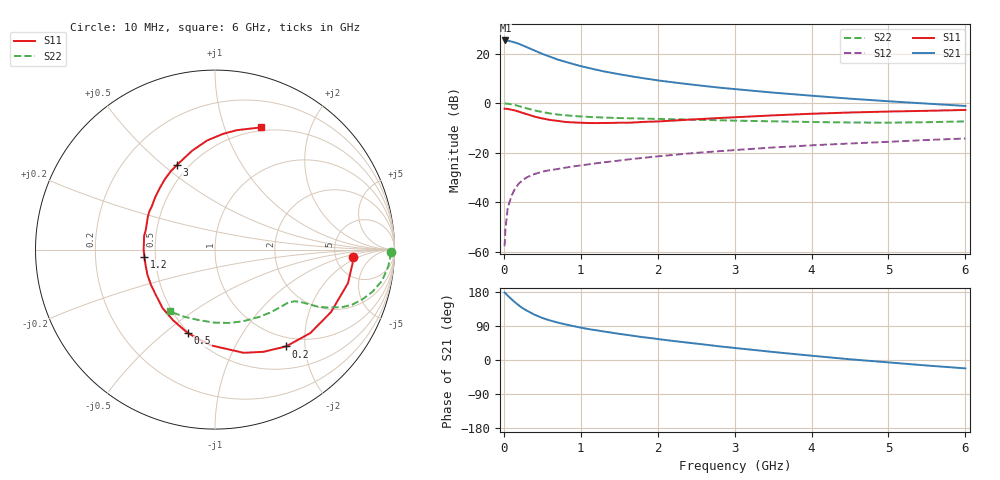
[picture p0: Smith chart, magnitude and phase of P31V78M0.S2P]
! SIEMENS Small Signal Semiconductors
! BFP181
! Si NPN RF Bipolar Junction Transistor in SOT143
! VCE = 1.75 V  IC = 8 mA
! Common Emitter S-Parameters:  March  1996
# GHz  S  MA  R  50
!  f  S11  S21  S12  S22
! GHz  MAG  ANG  MAG  ANG  MAG  ANG  MAG  ANG
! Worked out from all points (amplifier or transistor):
!   36 points, 10 MHz to 6 GHz, reference 50 ohm
!   highest |S21| = 25.3 dB at 20 MHz (marker M1)
!   |S21| within 3 dB of that: start of sweep to 320.8 MHz
!   unconditionally stable (mu >= 1): 1.112 GHz to end of sweep
!   at 250 MHz: K = 0.32, MSG = 27.1 dB, |S12| = -31.0 dB
!   at 1.4 GHz: K = 1.10, MAG = 15.9 dB, |S12| = -23.6 dB
!   at 6 GHz: K = 1.04, MAG = 5.4 dB, |S12| = -14.3 dB
!   S11 on the Smith chart (normalised r, x): 10 MHz: 7.31, -1.48; 200 MHz: 0.84, -1.64; 500 MHz: 0.49, -0.60; 1.2 GHz: 0.43, -0.04; 3 GHz: 0.43, +0.56; 6 GHz: 0.46, +1.34
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0.01  0.7678 -3.1  18.34 178.0  0.0013 75.6  0.9793 -0.9
0.02  0.7703 -5.8  18.35 176.4  0.0028 82.2  0.9782 -2.1
0.05  0.764 -14.2  18.19 169.9  0.0076 83.4  0.9701 -5.5
0.1  0.734 -28.3  17.43 160.4  0.0135 74.6  0.9464 -10.6
0.15  0.706 -41.2  16.59 151.4  0.0194 69.3  0.9083 -15.0
0.2  0.6689 -53.8  15.61 143.3  0.0243 64.8  0.8664 -18.7
0.25  0.6303 -64.6  14.43 136.0  0.0282 60.8  0.823 -21.9
0.3  0.5967 -74.5  13.42 130.2  0.0319 57.0  0.7818 -24.1
0.4  0.5337 -92.6  11.47 119.4  0.0371 52.1  0.7126 -27.0
0.5  0.4896 -108.0  9.828 111.0  0.0413 49.1  0.6591 -28.9
0.6  0.4576 -120.8  8.635 104.4  0.0445 47.5  0.6188 -29.9
0.7  0.4377 -131.8  7.559 98.8  0.0468 46.6  0.5886 -30.6
0.9  0.408 -150.4  6.148 89.7  0.0528 45.7  0.5513 -31.8
1.1  0.3964 -167.2  5.125 81.6  0.0582 45.1  0.5265 -33.2
1.2  0.3952 -174.0  4.713 78.5  0.061 45.3  0.5187 -34.1
1.7  0.4073 158.9  3.383 63.4  0.0755 45.3  0.4914 -39.3
2.2  0.4433 138.6  2.623 50.3  0.09 43.7  0.4724 -46.0
3  0.5173 114.2  1.918 31.8  0.1129 39.6  0.4426 -59.2
3.5  0.5655 103.0  1.627 21.2  0.1272 36.4  0.4287 -68.9
4.5  0.6461 86.1  1.229 1.9  0.1532 29.2  0.4065 -91.2
5.5  0.699 74.4  0.977 -14.6  0.1802 22.5  0.4118 -114.7
6  0.7277 69.3  0.877 -22.1  0.1932 18.5  0.4269 -126.4
